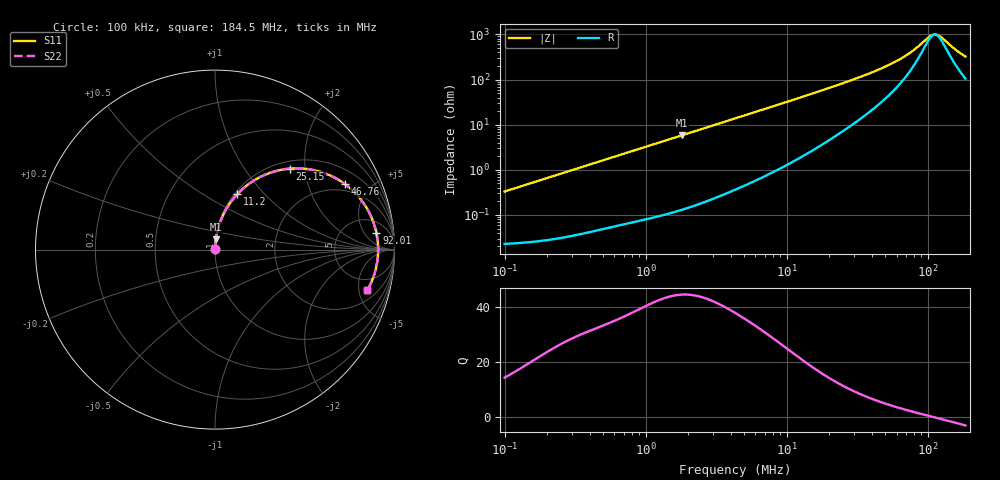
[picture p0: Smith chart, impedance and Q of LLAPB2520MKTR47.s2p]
! LLAPB2520MKTR47  S-PARAMETER MODEL  ( General Type )
! Model Generated by TAIYO YUDEN Corporation (http://www.ty-top.com)
! Version 1.0
! TAIYO YUDEN Control No. 151211NG33SB-FKC
! Copyright(c) 2015 TAIYO YUDEN CO.,LTD. All Rights Reserved.
! Product Description (link to TY-COMPAS)
! https://ds.yuden.co.jp/TYCOMPAS/or/detail?pn=LLAPB2520MKTR47M&u=M
! Products Name : Inductors
! Characteristics :
!  Inductance : 0.47 uH , SRF(min) : -Hz , DC Resistance(max) : 0.026 Ohm
!  Rated Current : Saturation :5800 mA , Temp Rise : 4100 mA (40 degC)
!  Case Size : 2.5 x 2.0 / 0.098 x 0.079 [mm/inch] , Thickness : 1.2 / 0.047 [mm/inch]
!  (Conditions: Temperature = 25 degC , DC Bias Current/Voltage = 0A / 0V)
! External Node Assignments :
!  1  o---GGG---o  2
! GND o---------o GND
! Frequency Range : 0.1MHz  -  184.468258MHz  [ 402 STEP ]
# MHz S RI R 50
! Freq[MHz].  S11 Real  S11 Imag  S21 Real  S21 Imag  S12 Real  S12 Imag  S22 Real  S22 Imag
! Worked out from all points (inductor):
!   401 points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, 100 kHz to 184.5 MHz, reference 50 ohm
!   read as one part in series: L = 525 nH near 103.8 kHz
!   highest Q = 44.7 at 1.809 MHz (marker M1), where L = 511 nH
!   self-resonance near 112.2 MHz
!   S11 on the Smith chart (normalised r, x): 100 kHz: 1.00, +0.01; 11.2 MHz: 1.03, +0.72; 25.15 MHz: 1.15, +1.66; 46.76 MHz: 1.63, +3.47; 92.01 MHz: 10, +10; 184.5 MHz: 3.10, -6.13
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0.1  0.000239 0.0033  0.9998 -0.0033  0.9998 -0.0033  0.000239 0.0033
0.352405  0.000514 0.0115  0.9995 -0.0115  0.9995 -0.0115  0.000514 0.0115
1.241892  0.00253 0.0399  0.9975 -0.0399  0.9975 -0.0399  0.00253 0.0399
1.808755  0.00465 0.0577  0.9954 -0.0577  0.9954 -0.0577  0.00465 0.0577
4.294977  0.0218 0.1336  0.9782 -0.1336  0.9782 -0.1336  0.0218 0.1336
7.408668  0.0594 0.2204  0.9406 -0.2204  0.9406 -0.2204  0.0594 0.2204
11.20381  0.1241 0.3089  0.8759 -0.3089  0.8759 -0.3089  0.1241 0.3089
15.13571  0.2047 0.3772  0.7953 -0.3772  0.7953 -0.3772  0.2047 0.3772
19.32614  0.2959 0.4239  0.7041 -0.4239  0.7041 -0.4239  0.2959 0.4239
25.14504  0.4177 0.4514  0.5823 -0.4514  0.5823 -0.4514  0.4177 0.4514
33.96951  0.5713 0.438  0.4287 -0.438  0.4287 -0.438  0.5713 0.438
46.76177  0.7223 0.3663  0.2777 -0.3663  0.2777 -0.3663  0.7223 0.3663
53.33896  0.774 0.3224  0.226 -0.3224  0.226 -0.3224  0.774 0.3224
72.05787  0.8614 0.2017  0.1386 -0.2017  0.1386 -0.2017  0.8614 0.2017
80.66224  0.8826 0.1518  0.1174 -0.1518  0.1174 -0.1518  0.8826 0.1518
92.00764  0.8994 0.0919  0.1006 -0.0919  0.1006 -0.0919  0.8994 0.0919
104.9488  0.9078 0.0309  0.0922 -0.0309  0.0922 -0.0309  0.9078 0.0309
111.0381  0.9089 0.00468  0.0911 -0.00468  0.0911 -0.00468  0.9089 0.00468
115.2926  0.9087 -0.0128  0.0913 0.0128  0.0913 0.0128  0.9087 -0.0128
124.297  0.9064 -0.0478  0.0936 0.0478  0.0936 0.0478  0.9064 -0.0478
161.7216  0.8768 -0.1681  0.1232 0.1681  0.1232 0.1681  0.8768 -0.1681
184.4683  0.8491 -0.2255  0.1509 0.2255  0.1509 0.2255  0.8491 -0.2255
